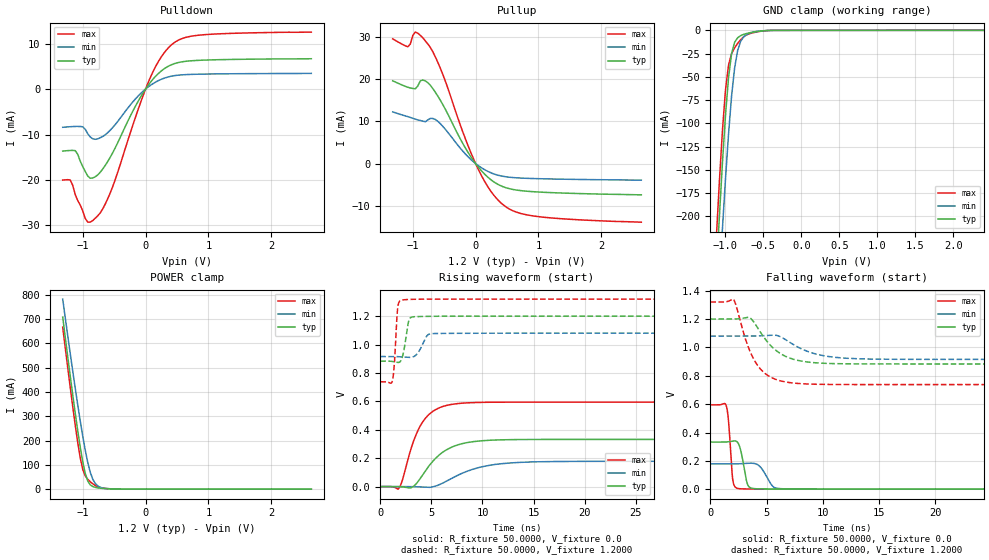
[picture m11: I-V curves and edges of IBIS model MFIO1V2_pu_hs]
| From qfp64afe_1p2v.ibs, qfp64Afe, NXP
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[Model] MFIO1V2_pu_hs
|   Model MFIO1V2_pu_hs
| This model was characterised for following simulation conditions:
| External (pad) voltage:
|   - Typ: 1.2V,   - Min: 1.08V,   - Max: 1.32V
| Library cells for typ/min/max conditions are connected as defined below:
|  IO - External Pad
|  A - Core Input
|  EN - Output Buffer Enable
|  BOOST - vdde
|  EHS - vdd
|  ENZI - vdd
|  EPD - gnd
|  EPUN - gnd
|  ZI - NC
|  ZIF - NC
|  gnd - gnd
|  gnde - gnde
|  vdd - vdd
|  vdde - vdde
| All other pins connected to ground
Model_type I/O
Polarity   Non-Inverting
Enable   Active-Low
Vinl =   0.3600V
Vinh =   0.8400V
Vmeas =  0.6000V
Cref =   20.0000F
Rref =   1.0000M
Vref =   0.0V
C_comp   1.6368pF   1.5495pF   1.7160pF
|C_comp_pullup   0.8278pF   0.8638pF   0.7802pF
|C_comp_pulldown   0.5961pF   0.6350pF   0.5601pF
[Model Spec]
| variable   typ   min   max
Vinh   0.3600V   0.3240V   0.3960V
Vinl   0.8400V   0.7560V   0.9240V
Vmeas   0.6000V   0.5400V   0.6600V
[Temperature Range]   25.0000   0.1250k   -40.0000
[Voltage Range]   1.2000V   1.0800V   1.3200V
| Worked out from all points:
|   slope of the pulldown table from 0 to 0.18 V, typ, clamps not added: 58.2 ohm
|   slope of the pullup table from 0 to 0.18 V, typ, clamps not added: 59.4 ohm
|   GND clamp passes 1 mA (typ) near -0.56 V on its own axis
|   POWER clamp passes 1 mA (typ) near -0.54 V on its own axis
|   rising waveform, R_fixture 50.0000, V_fixture 0.0: 20-80 % time 2.65ns typ, 3.74ns min, 1.91ns max; typ from 0.001 V to 0.332 V
|   rising waveform, R_fixture 50.0000, V_fixture 1.2000: 20-80 % time 419ps typ, 688ps min, 270ps max; typ from 0.883 V to 1.2 V
|   falling waveform, R_fixture 50.0000, V_fixture 0.0: 20-80 % time 471ps typ, 799ps min, 304ps max; typ from 0.332 V to 0.001 V
|   falling waveform, R_fixture 50.0000, V_fixture 1.2000: 20-80 % time 2.23ns typ, 2.81ns min, 1.78ns max; typ from 1.2 V to 0.883 V
[Pulldown]
|Voltage   I(typ)   I(min)   I(max)
-1.32V    -13.65mA   -8.413mA   -20.02mA
-1.2V     -13.51mA   -8.286mA   -20.01mA
-1.12V    -13.55mA   -8.228mA   -23.23mA
-920mV    -19.16mA   -9.85mA    -29.29mA
-720mV    -18.27mA   -10.7mA    -27.21mA
-520mV    -13.92mA   -8.406mA   -21.33mA
-160mV    -3.727mA   -2.148mA   -6.154mA
80mV      1.535mA    840.4uA    2.681mA
280mV     4.299mA    2.312mA    7.674mA
480mV     5.684mA    2.989mA    10.42mA
960mV     6.383mA    3.3mA      11.99mA
2.64V     6.671mA    3.446mA    12.53mA
[Pullup]
|Voltage   I(typ)   I(min)   I(max)
-1.32V    19.64mA    12.26mA    29.6mA
-1.08V    18.12mA    11.13mA    27.73mA
-960mV    17.74mA    10.54mA    31.21mA
-840mV    19.83mA    10.07mA    29.84mA
-720mV    18.57mA    10.71mA    27.56mA
-520mV    13.94mA    8.794mA    21.09mA
-200mV    4.663mA    2.883mA    7.362mA
40mV      -771.3uA   -452.7uA   -1.28mA
240mV     -3.804mA   -2.171mA   -6.507mA
480mV     -5.732mA   -3.143mA   -10.26mA
1.04V     -6.794mA   -3.614mA   -12.68mA
2.64V     -7.439mA   -3.951mA   -13.93mA
[GND_clamp]
|Voltage   I(typ)   I(min)   I(max)
-1.32V    -596.2mA   -647.7mA   -564.2mA
-1.12V    -261.8mA   -329.6mA   -222.9mA
-1.08V    -200.1mA   -270.2mA   -162.2mA
-1.04V    -142.5mA   -213.4mA   -108mA
-1V       -91.69mA   -160.1mA   -64.43mA
-960mV    -51.28mA   -111.9mA   -37.39mA
-920mV    -25.2mA    -71.06mA   -25.22mA
-880mV    -12.91mA   -40.7mA    -18.88mA
-800mV    -5.723mA   -11.8mA    -10.08mA
-680mV    -2.609mA   -2.945mA   -3.568mA
-440mV    -184.2uA   -204.3uA   -227.8uA
2.64V     0A         0A         0A
[POWER_clamp]
|Voltage   I(typ)   I(min)   I(max)
-1.32V    708.1mA    782.2mA    666.5mA
-1.2V     465.4mA    558mA      418.6mA
-1.12V    311.6mA    414.7mA    262.8mA
-1.04V    171.5mA    279.6mA    128mA
-1V       111.6mA    216.9mA    80.27mA
-960mV    64.04mA    159.3mA    53.84mA
-920mV    33mA       108.8mA    40.21mA
-880mV    17.41mA    68.43mA    30.39mA
-840mV    10.75mA    40.17mA    22.03mA
-760mV    5.272mA    13.2mA     9.331mA
-440mV    212.2uA    284.9uA    247uA
2.64V     0A         0A         0A
[Ramp]
| variable   typ   min   max
dV/dt_r  0.1992/2.6514n   0.1068/3.7358n   0.3565/1.9143n
dV/dt_f  0.1901/2.2311n   98.6074m/2.8135n   0.3492/1.7752n
R_load = 50.0000
[Rising Waveform]
R_fixture= 50.0000
V_fixture= 0.0
V_fixture_min= 0.0
V_fixture_max= 0.0
|time   V(typ)   V(min)   V(max)
0s        575.5uV    578.6uV    543.8uV
1.832ns   447.9uV    658.2uV    -10.14mV
2.125ns   -1.021mV   656.8uV    37.04mV
3.398ns   11.6mV     -173.7uV   348.3mV
4.656ns   135.7mV    -4.537mV   500.9mV
6.022ns   238.1mV    21.99mV    561.8mV
7.927ns   301.1mV    91.86mV    587.2mV
11.26ns   328.3mV    156.6mV    594.3mV
16.15ns   332.5mV    176.2mV    594.8mV
100ns     332.5mV    178.6mV    594.8mV
[Rising Waveform]
R_fixture= 50.0000
V_fixture= 1.2000
V_fixture_min= 1.0800
V_fixture_max= 1.3200
|time   V(typ)   V(min)   V(max)
0s        883.2mV    915.7mV    738.1mV
1.161ns   881.3mV    915.9mV    739.1mV
1.36ns    878.7mV    916.1mV    847.5mV
1.737ns   873.8mV    914.8mV    1.274V
2.12ns    904mV      913mV      1.313V
2.479ns   1.032V     911.2mV    1.316V
2.885ns   1.183V     909.7mV    1.318V
4.01ns    1.198V     981.7mV    1.319V
5.582ns   1.199V     1.078V     1.32V
100ns     1.2V       1.08V      1.32V
[Falling Waveform]
R_fixture= 50.0000
V_fixture= 0.0
V_fixture_min= 0.0
V_fixture_max= 0.0
|time   V(typ)   V(min)   V(max)
0s        332.5mV    178.6mV    594.8mV
1.419ns   332.9mV    178.5mV    589.4mV
1.619ns   334.8mV    178.5mV    484.4mV
2.015ns   339.9mV    178.4mV    59.26mV
2.682ns   281.8mV    180mV      3.336mV
3.316ns   34.03mV    182.9mV    1.74mV
4.19ns    2.916mV    174mV      1.044mV
5.596ns   1.26mV     17.54mV    689.5uV
6.705ns   887.2uV    2.446mV    602.5uV
100ns     575.5uV    578.6uV    543.8uV
[Falling Waveform]
R_fixture= 50.0000
V_fixture= 1.2000
V_fixture_min= 1.0800
V_fixture_max= 1.3200
|time   V(typ)   V(min)   V(max)
0s        1.2V       1.08V      1.32V
2.054ns   1.2V       1.08V      1.34V
2.276ns   1.2V       1.08V      1.3V
3.492ns   1.21V      1.08V      979.5mV
4.415ns   1.113V     1.081V     851.5mV
5.905ns   974.4mV    1.085V     772mV
7.934ns   906.1mV    996.5mV    745.1mV
10.45ns   887.1mV    936.6mV    739mV
15.34ns   883.3mV    916.7mV    738mV
100ns     883.2mV    915.7mV    738.1mV
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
